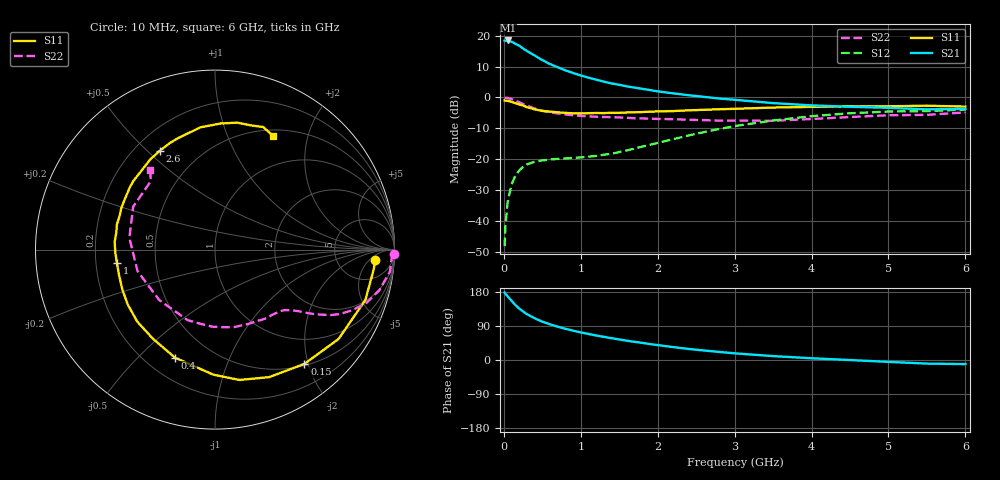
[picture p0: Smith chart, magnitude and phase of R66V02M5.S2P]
! SIEMENS Small Signal Semiconductors
! BFR193
! Si NPN RF Bipolar Junction Transistor in SOT23
! VCE = 6 V  IC = 2.5 mA
! Common Emitter S-Parameters:  May  1996
# GHz  S  MA  R  50
!  f  S11  S21  S12  S22
! GHz  MAG  ANG  MAG  ANG  MAG  ANG  MAG  ANG
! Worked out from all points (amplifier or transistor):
!   36 points, 10 MHz to 6 GHz, reference 50 ohm
!   highest |S21| = 18.5 dB at 50 MHz (marker M1)
!   |S21| within 3 dB of that: start of sweep to 273.8 MHz
!   unconditionally stable (mu >= 1): 1.099 GHz to 2.022 GHz
!   at 250 MHz: K = 0.26, MSG = 19.2 dB, |S12| = -22.5 dB
!   at 1.4 GHz: K = 1.10, MAG = 9.5 dB, |S12| = -18.2 dB
!   at 6 GHz: K = 0.99, MSG = 0.1 dB, |S12| = -3.9 dB
!   S11 on the Smith chart (normalised r, x): 10 MHz: 13, -8; 150 MHz: 0.53, -1.94; 400 MHz: 0.32, -0.65; 1 GHz: 0.29, -0.06; 2.6 GHz: 0.30, +0.55; 6 GHz: 0.57, +1.47
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0.01  0.8942 -3.8  8.339 177.8  0.0039 87.8  0.9963 -1.4
0.02  0.8911 -7.2  8.278 175.0  0.0082 88.9  0.9854 -2.8
0.05  0.8836 -18.5  8.381 167.7  0.0204 80.6  0.9825 -7.2
0.1  0.8496 -35.9  7.987 156.3  0.039 71.6  0.9429 -13.9
0.15  0.8083 -52.0  7.426 144.9  0.0544 63.1  0.8945 -19.4
0.2  0.7719 -67.0  6.899 135.8  0.0658 56.8  0.8367 -23.8
0.25  0.739 -79.4  6.206 127.9  0.0749 51.2  0.7842 -27.2
0.3  0.6967 -90.8  5.646 121.0  0.0823 47.5  0.7412 -29.5
0.4  0.642 -110.3  4.787 110.2  0.0909 41.8  0.6636 -32.9
0.5  0.6052 -124.8  4.024 101.2  0.0954 38.7  0.6091 -35.1
0.6  0.5906 -137.1  3.48 94.2  0.099 37.1  0.5762 -36.5
0.8  0.5624 -156.5  2.746 82.3  0.1028 37.4  0.5309 -39.5
1  0.5518 -172.0  2.27 72.8  0.107 41.4  0.5028 -42.8
1.1  0.5558 -178.5  2.091 68.7  0.1099 43.8  0.4941 -45.1
1.3  0.5581 170.3  1.802 61.1  0.1181 48.8  0.4822 -49.2
1.6  0.5709 156.1  1.511 50.8  0.1384 56.3  0.4688 -56.9
2.2  0.6014 132.7  1.166 34.1  0.2106 62.4  0.4451 -75.9
2.6  0.6304 119.2  1.023 25.1  0.2743 60.3  0.4297 -92.0
3.5  0.6861 96.7  0.81 10.3  0.4236 46.3  0.4191 -137.8
4.5  0.718 80.0  0.706 -0.1  0.5546 26.5  0.4814 172.2
5.5  0.7338 68.5  0.641 -9.5  0.6017 7.4  0.5223 133.4
6  0.7113 63.0  0.654 -10.8  0.6368 2.1  0.573 128.9
